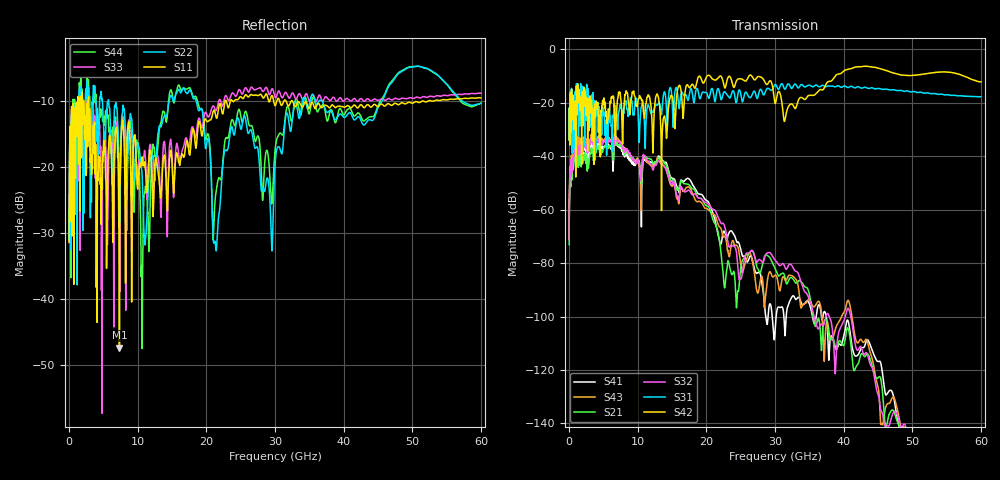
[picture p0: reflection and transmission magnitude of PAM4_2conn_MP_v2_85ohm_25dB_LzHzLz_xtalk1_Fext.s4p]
! Info: Touchstone file created by Circ.  Input file=FAB50GbE_2conn_Midplane_Examax_Topo2_v2_85ohm_25dB_LzHzLz.circ
# Hz S RI R 50
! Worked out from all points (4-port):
!   6000 points, 10 MHz to 60 GHz, reference 50 ohm
!   strongest paths, dB at 10 MHz, 15.01 GHz, 30.01 GHz, 45.01 GHz, 60 GHz:
!     S42: -34.0, -17.4, -20.2, -7.0, -12.1
!     S31: -33.9, -18.9, -13.1, -14.6, -17.7
!     S32: -71.2, -50.5, -78.9, -129.1, -165.4
!     S21: -73.1, -49.2, -81.9, -122.9, -157.6
!     S43: -70.7, -51.3, -84.5, -126.3, -169.3
!     S41: -69.2, -48.2, -105.9, -116.8, -169.7
!   lowest |S11| = -47.4 dB at 7.34 GHz (marker M1), VSWR 1.01, Z = 49.7 - j0.262 ohm
!   |S11| at or under -10 dB: start of sweep to 1.243 GHz; 2.846 GHz to 22.73 GHz (19.88 GHz wide, 155 % of centre); 32.57 GHz to 51.37 GHz (18.8 GHz wide, 44.8 % of centre)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
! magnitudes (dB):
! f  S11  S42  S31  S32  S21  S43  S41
! 10 MHz  -31.4  -34.0  -33.9  -71.2  -73.1  -70.7  -69.2
! 1.01 GHz  -10.9  -19.4  -15.3  -35.5  -38.4  -33.0  -35.0
! 7.34 GHz  -47.4  -16.2  -21.8  -34.5  -35.5  -33.9  -36.0
! 10.65 GHz  -18.4  -18.9  -19.5  -42.6  -45.8  -42.5  -47.4
! 13.6 GHz  -20.6  -29.9  -21.0  -43.3  -41.6  -43.0  -41.5
! 22.57 GHz  -11.0  -13.5  -15.9  -65.5  -87.8  -70.0  -68.0
! 60 GHz  -9.5  -12.1  -17.7  -165.4  -157.6  -169.3  -169.7
